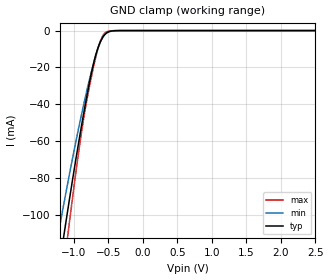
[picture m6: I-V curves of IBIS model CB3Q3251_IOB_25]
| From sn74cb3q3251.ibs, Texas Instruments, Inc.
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[Model]   CB3Q3251_IOB_25
Model_type  Terminator
| variable   typ   min   max
C_comp   16.85pF   13.20pF   20.46pF
| C_tri-state   16.85pF   13.20pF   20.46pF
[Temperature Range]   40   100   -40
| Ambient temperature   25   85   -40
[Voltage range]   2.5   2.3   2.7
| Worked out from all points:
|   GND clamp passes 1 mA (typ) near -0.51 V on its own axis
[GND Clamp]
| CB3Q3251_IOB_25
|   Voltage   I(typ)   I(min)   I(max)
-5.5V     -1.586A    -1.323A    -1.877A
-1.225V   -130.9mA   -110mA     -154.2mA
-1.13V    -107.2mA   -90.66mA   -123.6mA
-1.1V     -99.88mA   -84.71mA   -114.4mA
-1.065V   -91.48mA   -77.85mA   -103.8mA
-910mV    -55.89mA   -49.02mA   -60.27mA
-775mV    -28.13mA   -26.47mA   -30.31mA
-705mV    -16.2mA    -16.25mA   -17.78mA
-645mV    -8.66mA    -8.981mA   -8.813mA
-590mV    -4.087mA   -4.193mA   -3.371mA
-535mV    -1.521mA   -1.547mA   -900.4uA
2.5V      411.1pA    1.548nA    78.63pA
